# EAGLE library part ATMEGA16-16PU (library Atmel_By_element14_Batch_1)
Microcontroller
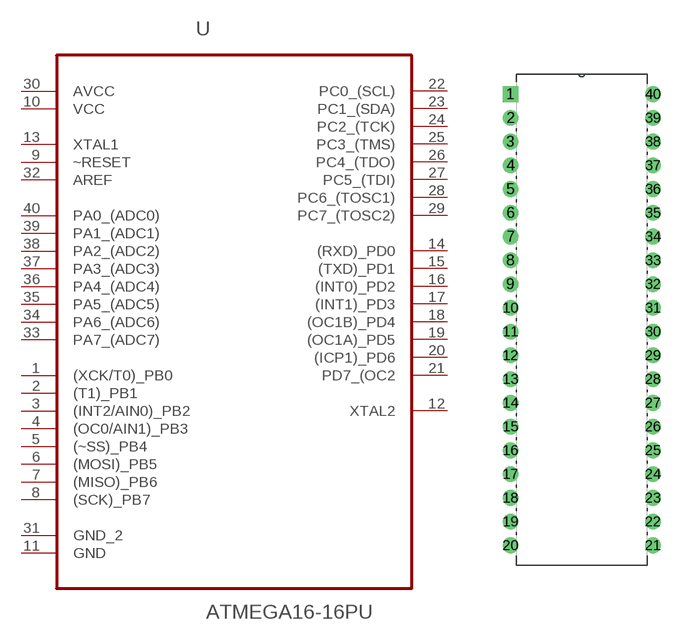
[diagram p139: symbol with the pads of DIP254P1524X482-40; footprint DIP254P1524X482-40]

Designator prefix U

## ATMEGA16-16PU (DESCRIPTION: Microcontroller; MPN: ATMEGA16-16PU; OC_FARNELL: 9171142; OC_NEWARK: 01M6885; PACKAGE: DIP-40; SUPPLIER: Atmel)  [DIP254P1524X482-40]
1  (XCK/T0)_PB0
2  (T1)_PB1
3  (INT2/AIN0)_PB2
4  (OC0/AIN1)_PB3
5  (~SS)_PB4
6  (MOSI)_PB5
7  (MISO)_PB6
8  (SCK)_PB7
9  ~RESET  in
10  VCC  pwr
11  GND  pas
12  XTAL2  out
13  XTAL1  in
14  (RXD)_PD0
15  (TXD)_PD1
16  (INT0)_PD2
17  (INT1)_PD3
18  (OC1B)_PD4
19  (OC1A)_PD5
20  (ICP1)_PD6
21  PD7_(OC2
22  PC0_(SCL)
23  PC1_(SDA)
24  PC2_(TCK)
25  PC3_(TMS)
26  PC4_(TDO)
27  PC5_(TDI)
28  PC6_(TOSC1)
29  PC7_(TOSC2)
30  AVCC  pwr
31  GND_2  pas
32  AREF  in
33  PA7_(ADC7)
34  PA6_(ADC6)
35  PA5_(ADC5)
36  PA4_(ADC4)
37  PA3_(ADC3)
38  PA2_(ADC2)
39  PA1_(ADC1)
40  PA0_(ADC0)

## Footprint DIP254P1524X482-40 (pad centres in mm)
drill 1.118 square: 1 -15.24,48.26
drill 1.118: 2 -15.24,45.72; 3 -15.24,43.18; 4 -15.24,40.64; 5 -15.24,38.1; 6 -15.24,35.56; 7 -15.24,33.02; 8 -15.24,30.48; 9 -15.24,27.94; 10 -15.24,25.4; 11 -15.24,22.86; 12 -15.24,20.32; 13 -15.24,17.78; 14 -15.24,15.24; 15 -15.24,12.7; 16 -15.24,10.16; 17 -15.24,7.62; 18 -15.24,5.08; 19 -15.24,2.54; 20 -15.24,0; 21 0,0; 22 0,2.54; 23 0,5.08; 24 0,7.62; 25 0,10.16; 26 0,12.7; 27 0,15.24; 28 0,17.78; 29 0,20.32; 30 0,22.86; 31 0,25.4; 32 0,27.94; 33 0,30.48; 34 0,33.02; 35 0,35.56; 36 0,38.1; 37 0,40.64; 38 0,43.18; 39 0,45.72; 40 0,48.26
